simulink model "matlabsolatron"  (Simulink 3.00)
settings: Solver=ode1  SolverMode=SingleTasking  StartTime=0.0  StopTime=inf  RelTol=1e-3
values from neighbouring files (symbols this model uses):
  h = 0.01    [design.m]    (also in initfra.m; initlab1.m; tst.m)
undefined symbols (not defined in the file or in its folder): bias, h_fra, Tstart, Tstop, u0, w

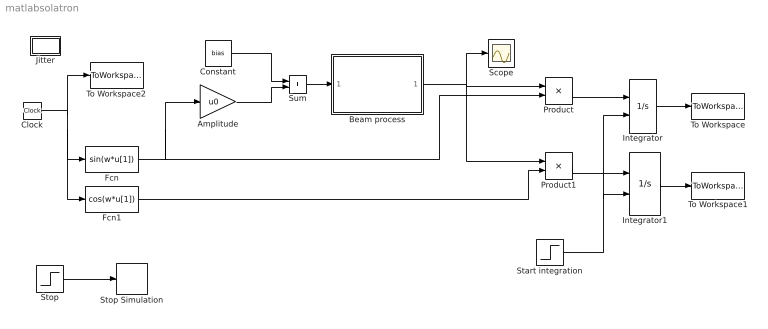
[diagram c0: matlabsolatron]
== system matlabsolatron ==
  Amplitude : Gain  Gain=u0  SaturateOnIntegerOverflow=on
  Beam process : Subsystem
  Clock : Clock
  Constant : Constant  Value=bias
  Fcn : Fcn  Expr=sin(w*u[1])
  Fcn1 : Fcn  Expr=cos(w*u[1])
  Integrator : Integrator  ExternalReset=rising  InitialConditionSource=internal  InitialCondition=0  LimitOutput=off  UpperSaturationLimit=inf  LowerSaturationLimit=-inf  ShowSaturationPort=off  ShowStatePort=off  AbsoluteTolerance=auto
  Integrator1 : Integrator  ExternalReset=rising  InitialConditionSource=internal  InitialCondition=0  LimitOutput=off  UpperSaturationLimit=inf  LowerSaturationLimit=-inf  ShowSaturationPort=off  ShowStatePort=off  AbsoluteTolerance=auto
  Jitter : Subsystem
  Product : Product  Inputs=2  SaturateOnIntegerOverflow=on
  Product1 : Product  Inputs=2  SaturateOnIntegerOverflow=on
  Scope : Scope
  Start integration : Step  Time=Tstart  Before=0  After=1  SampleTime=h
  Stop : Step  Time=Tstop  Before=0  After=1  SampleTime=0
  Stop Simulation : Stop
  Sum : Sum  Inputs=++  SaturateOnIntegerOverflow=on
  To Workspace : ToWorkspace  VariableName=s_T  SampleTime=-1  SaveFormat=Matrix
  To Workspace1 : ToWorkspace  VariableName=c_T  SampleTime=-1  SaveFormat=Matrix
  To Workspace2 : ToWorkspace  VariableName=time  SampleTime=-1  SaveFormat=Matrix
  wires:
  Product/1 -> Integrator/1
  Product1/1 -> Integrator1/1
  Fcn1/1 -> Product1/2
  Integrator/1 -> To Workspace/1
  Integrator1/1 -> To Workspace1/1
  Clock/1 -> Fcn/1, Fcn1/1, To Workspace2/1
  Fcn/1 -> Product/2, Amplitude/1
  Sum/1 -> Beam process/1(In1)
  Amplitude/1 -> Sum/2
  Constant/1 -> Sum/1
  Start integration/1 -> Integrator1/2, Integrator/2
  Beam process/1(Out1) -> Product/1, Product1/1, Scope/1
  Stop/1 -> Stop Simulation/1

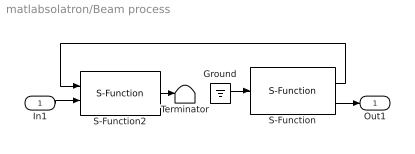
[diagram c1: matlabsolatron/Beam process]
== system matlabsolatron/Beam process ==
  In1 : Inport  Port=1  PortWidth=-1  SampleTime=-1  DataType=auto
  Ground : Ground
  S-Function : S-Function  FunctionName=analogin  Parameters=h_fra [0]  PortCounts=[]  SFunctionModules=''
  S-Function2 : S-Function  FunctionName=analogout  Parameters=h_fra [0]  PortCounts=[]  SFunctionModules=''
  Terminator : Terminator
  Out1 : Outport  Port=1
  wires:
  Ground/1 -> S-Function/1
  S-Function2/1 -> Terminator/1
  S-Function/1 -> S-Function2/1
  S-Function/2 -> Out1/1
  In1/1 -> S-Function2/2

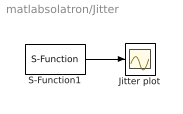
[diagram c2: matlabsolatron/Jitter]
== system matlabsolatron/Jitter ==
  Jitter plot : Scope
  S-Function1 : S-Function  FunctionName=timer  Parameters=h_fra  PortCounts=[]  SFunctionModules=''
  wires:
  S-Function1/1 -> Jitter plot/1
